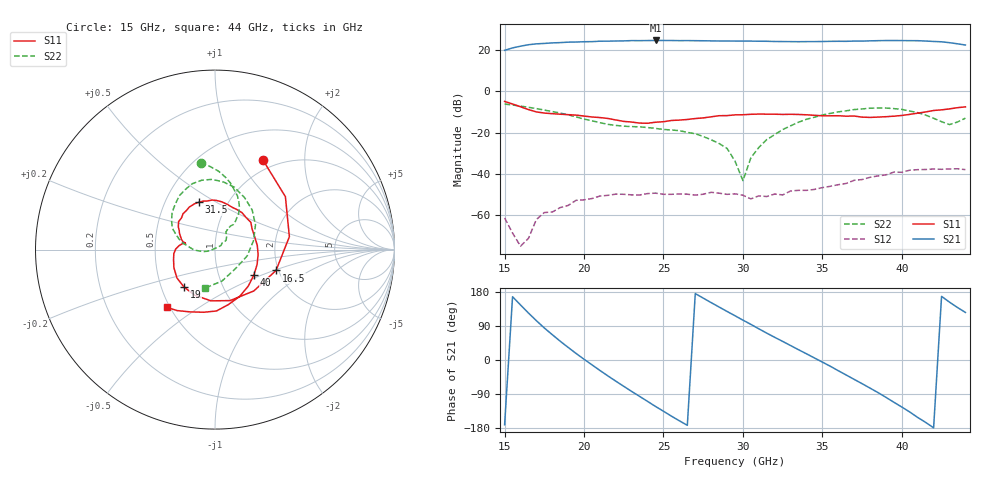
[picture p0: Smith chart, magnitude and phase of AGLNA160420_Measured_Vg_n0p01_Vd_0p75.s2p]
! Filename4Jim: AG10_M048_0403_Vg_n0p01_Vd_0p75_CP2_NF.s2p
! Calibration: TFN_AG02
! Notes: BK
! Row:4, Col:3
! Probes: GSG150
! Prober: TS150
! Date: 2024-01-12 13:15:04
! DC: Vg.V=-0.0112427, Vg.I=-1.41339e-09, Vd.V=0.750009, Vd.I=0.0347102
! Keysight Technologies,N5245B,MY58421923,A.15.75.19
! AGMDC-PNAX50 Fri Jan 12 13:15:48 2024
# HZ S DB R 50
!freq (Hz)  S11DB  S11A  S21DB  S21A  S12DB  S12A  S22DB  S22A
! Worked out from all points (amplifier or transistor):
!   59 points, 15 GHz to 44 GHz, reference 50 ohm
!   highest |S21| = 24.6 dB at 24.5 GHz (marker M1)
!   |S21| within 3 dB of that: 15.87 GHz to end of sweep
!   unconditionally stable (mu >= 1): start of sweep to end of sweep
!   at 19.5 GHz: K = 12.38, MAG = 24.4 dB, |S12| = -52.8 dB
!   at 29.5 GHz: K = 8.63, MAG = 24.7 dB, |S12| = -49.7 dB
!   at 44 GHz: K = 2.40, MAG = 23.6 dB, |S12| = -38.0 dB
!   lowest NFmin = 1.02 dB at 38.5 GHz
!   S11 on the Smith chart (normalised r, x): 15 GHz: 0.86, +1.27; 16.5 GHz: 1.94, -0.52; 19 GHz: 0.65, -0.29; 31.5 GHz: 0.73, +0.42; 40 GHz: 1.47, -0.45; 44 GHz: 0.48, -0.38
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1.5e10  -4.93 62.0  19.84 -170.9  -61.38 37.6  -6.21 99.4
1.55e10  -6.19 36.9  21.01 167.0  -68.72 17.8  -6.68 93.4
1.65e10  -8.89 -18.9  22.55 124.0  -71.32 -136.2  -7.78 82.0
1.75e10  -10.57 -73.5  23.18 84.5  -58.78 170.6  -9.13 72.1
1.9e10  -11.34 -129.6  23.80 33.2  -55.35 160.8  -11.40 59.5
2e10  -12.03 -155.9  24.01 1.9  -52.62 142.2  -13.49 55.3
2.1e10  -12.75 -174.4  24.27 -27.6  -50.79 130.0  -15.23 53.7
2.25e10  -14.61 170.1  24.42 -69.5  -49.95 106.3  -16.93 57.8
2.45e10  -15.00 166.5  24.62 -122.7  -49.38 80.6  -18.00 58.4
2.5e10  -14.77 166.4  24.61 -135.2  -49.94 70.4  -18.51 58.1
2.7e10  -13.22 155.2  24.51 175.3  -50.33 57.5  -20.58 46.6
2.95e10  -11.45 131.8  24.34 116.8  -49.71 11.6  -33.82 40.2
3.15e10  -11.09 108.9  24.23 70.9  -51.02 -32.2  -23.41 -170.6
3.3e10  -11.16 93.3  24.06 38.1  -48.33 -75.6  -16.74 174.1
3.45e10  -11.66 74.9  24.07 5.4  -47.58 -124.4  -12.57 158.4
3.6e10  -11.87 53.9  24.22 -28.3  -45.27 -152.0  -10.00 139.1
3.75e10  -12.53 29.1  24.31 -62.5  -42.79 -176.2  -8.57 116.7
3.95e10  -12.08 -19.6  24.58 -111.5  -39.17 147.1  -8.41 82.8
4e10  -11.74 -33.2  24.57 -124.2  -39.28 139.1  -8.78 72.7
4.1e10  -10.61 -62.2  24.51 -151.6  -38.00 119.3  -10.38 46.8
4.2e10  -9.32 -88.7  24.14 -179.0  -37.69 100.7  -13.10 13.5
4.4e10  -7.58 -129.5  22.42 125.6  -37.98 66.0  -13.05 -105.0
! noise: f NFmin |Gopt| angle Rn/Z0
1.5e+10  2.562  0  90  0.201
1.8e+10  2.011  0.04773  -57.6  0.2967
2.1e+10  1.726  0  90  0.122
2.45e+10  1.574  0.13  89.18  0.4727
2.75e+10  1.436  0.1122  -162.5  0.2055
3.1e+10  1.446  0.06567  -174  0.4191
3.4e+10  1.446  0.06446  -104.3  0.1571
3.75e+10  1.228  0  90  0.08169
4.05e+10  1.261  0.05364  12.21  0.7986
4.4e+10  1.616  0  90  0.1127
